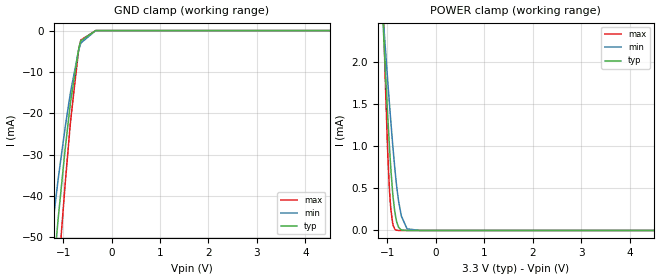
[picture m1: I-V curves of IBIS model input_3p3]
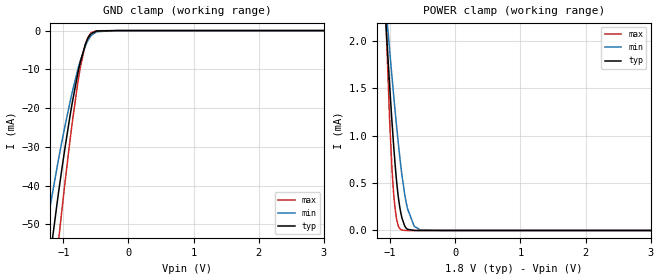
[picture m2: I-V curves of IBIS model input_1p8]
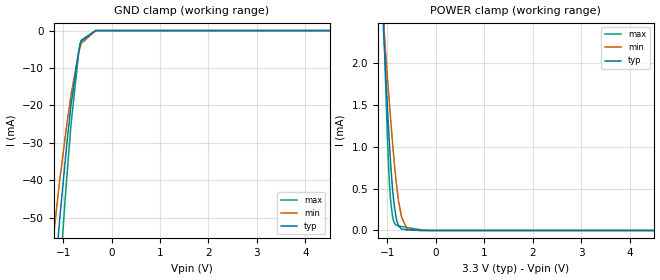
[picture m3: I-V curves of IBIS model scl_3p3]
|Texas Instruments Incorporated
|Low-Power Audio Codec With 1.3W Stereo Class-D Speaker Amplifier
| Marketing part#   Digital Voltage Range   Package-type   #pins
| TLV320AIC3110IRHBT   1.1V-3.6V   QFN   32
| TLV320AIC3110IRHBR   1.1V-3.6V   QFN   32
[IBIS Ver]   4.1
[File name]   tlv320aic3110.ibs
[File Rev]   1.0
[Date]   7/8/2013
[Source]
| Texas Instruments Incorporated.
| Analog-eLab Design Center, HPA
| 12500 TI Blvd
| Dallas, TX -75243
[Notes]   Revision History:
| Rev 1.0: 7/8/2013
| - Initial version of the model.Relative part of TLV320AIC3100
| - Model generated from simulations in TISPICE
| - Model matched to SPICE simulation
| - C_comp although listed in numerical order of value are
|   obtained from varying PVT conditions. For PVT conditions for
|   each specific value refer the buffer description under
|   respective [Model]. IBIS model user is responsible for using
|   appropriate C_comp to simulate for Signal Integrity.
[Disclaimer]
| This model is designed as an aid for customers of Texas Instruments.
| TI and its licensors and suppliers make no warranties, either expressed
| or implied, with respect to this  model, including the warranties of
| merchantability or fitness for a particular purpose. The model is
| provided solely on an "as is" basis. The entire risk as to its quality
| and performance is with the customer.
[Copyright]
(C) Copyright 2013 Texas Instruments Incorporated.All rights reserved.
|   TLV320AIC3110
[Component]   TLV320AIC3110
[Manufacturer]   TI
[Package]   |32 QFN   -  RHB package
|   typ   min   max
R_pkg   0.08098   0.06239   0.10488
L_pkg   1.16681nH   0.86338nH   1.56075nH
C_pkg   0.10772pF   0.08945pF   0.12937pF
[Pin]  signal_name   model_name   R_pin   L_pin   C_pin
1   IOVSS   gnd   0.10892   1.62955nH  0.14775pF
2   IOVDD   power   0.04653   1.07174nH  0.17671pF
3   DVDD   power   0.07771   1.11075nH  0.11419pF
4   DOUT   DOUT   0.07046   0.99253nH  0.10023pF
5   DIN   INPUT   0.06239   0.86338nH  0.09118pF
6   WCLK   IO   0.06314   0.87528nH  0.09150pF
7   BCLK   IO   0.07128   1.00585nH  0.09967pF
8   MCLK   INPUT   0.09352   1.37325nH  0.11994pF
9   SDA   SDA   0.10292   1.52935nH  0.12937pF
10   SCL   SCL   0.09432   1.38475nH  0.11902pF
11   VOL/MICDET   nc   0.10819   1.61825nH  0.13840pF
12   MICBIAS   nc   0.09648   1.42115nH  0.13125pF
13   MIC1LP   nc   0.09101   1.32875nH  0.12465pF
14   MIC1RP   nc   0.09181   1.34045nH  0.12548pF
15   MIC1LM   nc   0.09852   1.45105nH  0.13029pF
16   AVSS   gnd   0.10995   1.64175nH  0.13895pF
17   AVDD   power   0.10504   1.55835nH  0.13042pF
18   DVSS   gnd   0.08266   1.18695nH  0.10829pF
19   SPLM   nc   0.04210   0.95582nH  0.15152pF
20   SPLVSS   gnd   0.03571   0.74426nH  0.13884pF
21   SPLVDD   power   0.03284   0.65209nH  0.12329pF
22   SPLP   nc   0.03065   0.58402nH  0.11451pF
23   SPRM   nc   0.03448   0.70984nH  0.12743pF
24   SPRVDD   power   0.04322   0.95015nH  0.15314pF
25   SPRVSS   gnd   0.04598   1.11891nH  0.14352pF
26   SPRP   nc   0.04667   1.08878nH  0.15160pF
27   HPL   nc   0.09068   1.31875nH  0.12486pF
28   HPVDD   power   0.07560   1.07045nH  0.11000pF
29   HPVSS   gnd   0.06652   0.92471nH  0.09696pF
30   HPR   nc   0.06717   0.93728nH  0.09351pF
31   _RESET   INPUT   0.06590   0.91612nH  0.08945pF
32   GPIO1   IO   0.10488   1.56075nH  0.12918pF
33   thermal_pad   nc   0.00008   0.00125nH  0.48256pF
|   Model Selectors
[Model Selector] DOUT
dout_3p3  3.3V digital 3-state
dout_1p8  1.8V digital 3-state
[Model Selector] INPUT
input_3p3  3.3V digital input
input_1p8  1.8V digital input
[Model Selector] IO
io_3p3  3.3V digital I/O
io_1p8  1.8V digital I/O
[Model Selector] SDA
sda_3p3  3.3V digital I/O_open_drain
sda_1p8  1.8V digital I/O_open_drain
[Model Selector] SCL
scl_3p3  3.3V digital input
scl_1p8  1.8V digital input
| Models and submodels in the file (10): input_3p3 (Input), input_1p8 (Input), scl_3p3 (Input), scl_1p8 (Input), dout_3p3 (3-state), dout_1p8 (3-state), io_3p3 (I/O), io_1p8 (I/O), sda_3p3 (I/O_open_drain), sda_1p8 (I/O_open_drain)
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|   input_3p3 Model
[Model]   input_3p3
Model_type   Input
Vinl = 0.99
Vinh = 2.31
|   typ   min   max
|   (nom PVT)   (fast PVT)   (slow PVT)
C_comp   9.787e-13   9.710e-13   9.825e-13
[Model spec]
Vinl   0.99   0.90   1.08
Vinh   2.31   2.10   2.52
| Where nom  PVT is Nominal Process, 3.3V, 27C
|   Fast PVT is Strong Process,  3.6V, -40C
|   Slow PVT is Weak Process,   3V, 125C
[Voltage Range]   3.3   3   3.6
|Junction Temperature
[Temperature Range]   27   125   -40
[Power Clamp Reference]   3.3   3   3.6
[GND Clamp Reference]   0   0   0
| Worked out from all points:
|   POWER clamp passes 1 mA (typ) near -0.96 V on its own axis
[GND Clamp]
|   Voltage   I(typ)   I(min)   I(max)
-3.3V     -1.785A    -1.561A    -1.955A
-1.478V   -95.01mA   -72.56mA   -121.1mA
-1.1V     -45.05mA   -35.58mA   -58.51mA
-960.3mV  -28.73mA   -23.47mA   -37.2mA
-851.4mV  -17.55mA   -15.06mA   -22.27mA
-687mV    -4.837mA   -5.08mA    -5.214mA
-660mV    -3.469mA   -3.905mA   -3.489mA
-636mV    -2.471mA   -3.002mA   -2.294mA
-330mV    -959.6nA   -9.225uA   -101.1nA
6.6V      0A         0A         0A
[POWER Clamp]
|   Voltage   I(typ)   I(min)   I(max)
-3.3V     32.15mA    22.37mA    56.05mA
-1.096V   2.542mA    2.603mA    2.836mA
-1.043V   1.918mA    2.173mA    1.777mA
-993mV    1.361mA    1.779mA    925.2uA
-952.8mV  951.7uA    1.471mA    441uA
-927.6mV  723.2uA    1.284mA    249.7uA
-894.3mV  469.8uA    1.048mA    97.26uA
-822mV    139.6uA    596.6uA    5.164uA
-768mV    36.85uA    344.7uA    433.9nA
-714mV    6.429uA    178.6uA    35.81nA
-594mV    89.79nA    19.58uA    0A
6.6V      0A         0A         0A
|   input_1p8 Model
[Model]   input_1p8
Model_type   Input
Vinl = 0.54
Vinh = 1.26
|   typ   min   max
|   (nom PVT)   (fast PVT)   (slow PVT)
C_comp   1.043e-12   1.039e-12   1.047e-12
[Model spec]
Vinl   0.54   0.486   0.594
Vinh   1.26   1.134   1.386
| Where nom  PVT is Nominal Process, 1.8V, 27C
|   Fast PVT is Strong Process,  1.98V, -40C
|   Slow PVT is Weak Process,   1.62V, 125C
[Voltage Range]   1.8   1.62   1.98
|Junction Temperature
[Temperature Range]   27   125   -40
[Power Clamp Reference]   1.8   1.62   1.98
[GND Clamp Reference]   0   0   0
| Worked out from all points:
|   GND clamp passes 1 mA (typ) near -0.58 V on its own axis
|   POWER clamp passes 1 mA (typ) near -0.96 V on its own axis
[GND Clamp]
|   Voltage   I(typ)   I(min)   I(max)
-1.8V     -244.1mA   -134.4mA   -356.2mA
-1.319V   -73.19mA   -56.39mA   -94.04mA
-1.074V   -41.87mA   -33.23mA   -54.41mA
-1.028V   -36.37mA   -29.15mA   -47.25mA
-901.8mV  -22.52mA   -18.82mA   -28.94mA
-756.7mV  -9.431mA   -8.799mA   -11.3mA
-659.5mV  -3.448mA   -3.885mA   -3.461mA
-622.3mV  -1.992mA   -2.548mA   -1.754mA
-572.4mV  -796.9uA   -1.285mA   -556.1uA
-487.8mV  -109.3uA   -293.5uA   -47.67uA
-180mV    0A         -175.4nA   0A
3.6V      0A         0A         0A
[POWER Clamp]
|   Voltage   I(typ)   I(min)   I(max)
-1.8V     11.74mA    8.748mA    19.35mA
-1.075V   2.291mA    2.431mA    2.403mA
-1.058V   2.089mA    2.292mA    2.061mA
-1.004V   1.481mA    1.865mA    1.095mA
-972.4mV  1.145mA    1.619mA    648.1uA
-948.6mV  911.8uA    1.439mA    403.5uA
-901.8mV  521.3uA    1.1mA      123.2uA
-835.2mV  180.5uA    670.8uA    9.312uA
-732.4mV  12.01uA    226.7uA    83.64nA
-630.4mV  330.9nA    44.02uA    0A
-528.3mV  0A         3.71uA     0A
3.6V      0A         0A         0A
|   scl_3p3 Model
[Model]   scl_3p3
Model_type   Input
Vinl = 0.99
Vinh = 2.31
|   typ   min   max
|   (nom PVT)   (fast PVT)   (slow PVT)
C_comp   1.114e-12   1.105e-12   1.114e-12
| Where nom  PVT is Nominal Process, 3.3V, 27C
|   Fast PVT is Strong Process,  3.6V, -40C
|   Slow PVT is Weak Process,   3V, 125C
[Model spec]
Vinl   0.99   0.90   1.08
Vinh   2.31   2.10   2.52
[Voltage Range]   3.3   3   3.6
|Junction Temperature
[Temperature Range]   27   125   -40
[Power Clamp Reference]   3.3   3   3.6
[GND Clamp Reference]   0   0   0
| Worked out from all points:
|   POWER clamp passes 1 mA (typ) near -0.95 V on its own axis
[GND Clamp]
|   Voltage   I(typ)   I(min)   I(max)
-3.3V     -1.799A    -1.559A    -1.981A
-1.47V    -113.7mA   -86.89mA   -144.9mA
-1.09V    -53.03mA   -41.95mA   -68.9mA
-1.066V   -49.56mA   -39.38mA   -64.41mA
-937.2mV  -31.82mA   -26.19mA   -41.11mA
-841.2mV  -20.14mA   -17.39mA   -25.46mA
-678mV    -5.292mA   -5.667mA   -5.59mA
-653.4mV  -3.859mA   -4.421mA   -3.807mA
-632.4mV  -2.845mA   -3.494mA   -2.609mA
-330mV    -1.164uA   -11.12uA   -122.9nA
6.6V      0A         0A         0A
[POWER Clamp]
|   Voltage   I(typ)   I(min)   I(max)
-3.3V     32.44mA    22.56mA    56.44mA
-1.096V   2.591mA    2.619mA    2.932mA
-1.043V   1.961mA    2.185mA    1.866mA
-999.6mV  1.472mA    1.84mA     1.108mA
-963.6mV  1.093mA    1.56mA     627.4uA
-927.6mV  755.3uA    1.29mA     324.1uA
-882mV    420.9uA    968.9uA    132.5uA
-822mV    162.1uA    599.1uA    66.58uA
-702.9mV  17.31uA    153.9uA    47.23uA
-594mV    6.199uA    19.71uA    34.8uA
-330mV    249.7nA    22.98nA    9.678uA
6.6V      0A         0A         0A
